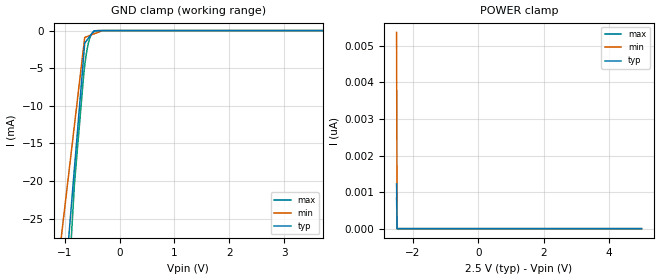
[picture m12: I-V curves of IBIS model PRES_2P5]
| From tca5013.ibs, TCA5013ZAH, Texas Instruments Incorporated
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[Model]   PRES_2P5
Model_type   Input
Vinl = .75
Vinh = 1.75
|   typ   min   max
C_comp   0.731p   0.503p   0.930p
[Model spec]
|subparameter
Vinl   0.75   0.675   0.825
Vinh   1.75   1.575   1.925
[Voltage Range]   2.5   2.25   2.75
[Temperature Range]   27   125   -40
[Power Clamp Reference]   2.5   2.25   2.75
[GND Clamp Reference]   0   0   0
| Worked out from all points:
|   GND clamp passes 1 mA (typ) near -0.56 V on its own axis
[GND Clamp]
|   Voltage   I(typ)   I(min)   I(max)
-2.5V     -204mA     -159mA     -266.1mA
-1.383V   -68.26mA   -47.62mA   -91.26mA
-820mV    -18.31mA   -12.59mA   -20.43mA
-647.5mV  -2.995mA   -1.844mA   -5.557mA
-632.5mV  -1.663mA   -909.5uA   -4.642mA
-610mV    -1.443mA   -846.7uA   -3.429mA
-587.5mV  -1.223mA   -783.9uA   -2.422mA
-557.5mV  -929.8uA   -700.2uA   -1.409mA
-520mV    -563.1uA   -595.6uA   -628.3uA
-467.5mV  -49.75uA   -449.1uA   -163.7uA
-306.9mV  -439.4nA   -1.188uA   -652nA
5V        0A         0A         0A
[POWER Clamp]
|   Voltage   I(typ)   I(min)   I(max)
-2.5V     1.225nA    5.366nA    843.3pA
-2.485V   0A         0A         0A
-512.5mV  0A         0A         0A
5V        0A         0A         0A
